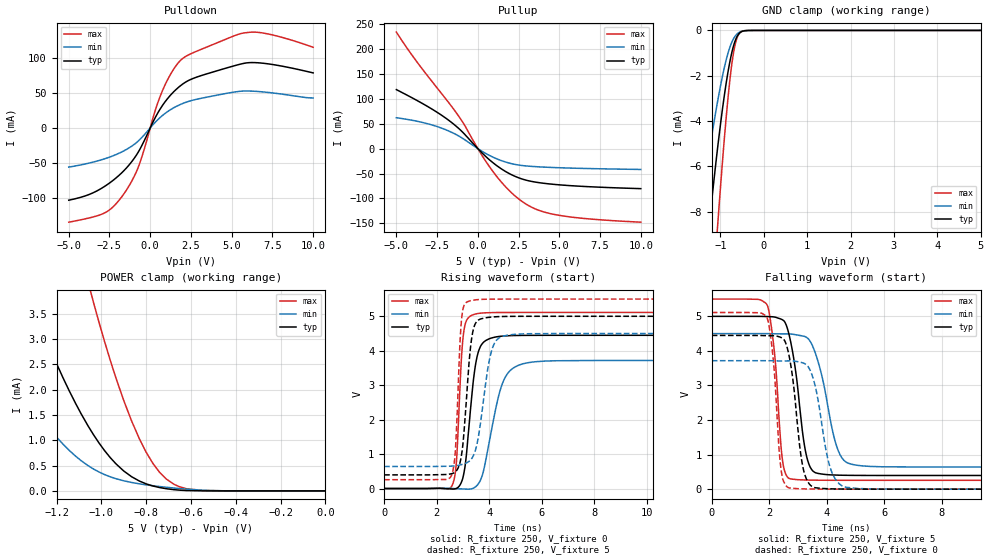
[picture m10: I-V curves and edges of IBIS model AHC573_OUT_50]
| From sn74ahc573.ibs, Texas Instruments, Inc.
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[Model]   AHC573_OUT_50
Model_type  3-state
Enable   Active-Low
Vref =   0.0
Rref =   1000
Cref =   50p
Vmeas =   2.5
| variable   typ   min   max
C_comp   2.10pF   1.84pF   2.26pF
| C_pullup   3.24pF   1.95pF   4.10pF
| C_pulldown   2.37pF   1.77pF   2.97pF
| C_tri-state   2.10pF   1.84pF   2.26pF
[Temperature Range]   40   100   -40
| Ambient temperature   25   85   -40
[Voltage range]   5   4.5   5.5
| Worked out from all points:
|   slope of the pulldown table from 0 to 0.75 V, typ, clamps not added: 23.5 ohm
|   slope of the pullup table from 0 to 0.75 V, typ, clamps not added: 32 ohm
|   GND clamp passes 1 mA (typ) near -0.74 V on its own axis
|   POWER clamp passes 1 mA (typ) near -1.02 V on its own axis
|   rising waveform, R_fixture 250, V_fixture 0: 20-80 % time 352ps typ, 620ps min, 198ps max; typ from 0 V to 4.45 V
|   falling waveform, R_fixture 250, V_fixture 5: 20-80 % time 427ps typ, 600ps min, 291ps max; typ from 5 V to 0.396 V
|   rising waveform, R_fixture 250, V_fixture 5: 20-80 % time 283ps typ, 440ps min, 176ps max; typ from 0.396 V to 5 V
|   falling waveform, R_fixture 250, V_fixture 0: 20-80 % time 363ps typ, 477ps min, 257ps max; typ from 4.45 V to 0 V
[GND Clamp]
| AHC573_OUT_50
|   Voltage   I(typ)   I(min)   I(max)
-5V       -113.4mA   -74.55mA   -144mA
-1.5V     -13.43mA   -8.541mA   -21.28mA
-1.27V    -8.795mA   -5.502mA   -14.35mA
-1.245V   -8.325mA   -5.193mA   -13.62mA
-1.07V    -5.258mA   -3.179mA   -8.755mA
-1.05V    -4.935mA   -2.968mA   -8.227mA
-875mV    -2.416mA   -1.357mA   -3.998mA
-765mV    -1.214mA   -649.6uA   -1.901mA
-665mV    -483.2uA   -264uA     -658.5uA
-615mV    -261.2uA   -152.9uA   -319.9uA
-545mV    -91.09uA   -61.69uA   -92.75uA
5V        41.61nA    4.678uA    381.8nA
[POWER Clamp]
| AHC573_OUT_50
|   Voltage   I(typ)   I(min)   I(max)
-5V       96.37mA    61.09mA    155.9mA
-1.595V   7.508mA    3.875mA    16.25mA
-1.32V    3.818mA    1.757mA    9.35mA
-1.2V     2.518mA    1.064mA    6.763mA
-1.06V    1.29mA     502uA      4.143mA
-1.035V   1.111mA    433.1uA    3.726mA
-935mV    536.6uA    242.1uA    2.235mA
-865mV    281uA      167.1uA    1.384mA
-800mV    139.6uA    120.4uA    765.1uA
-710mV    43.55uA    72.39uA    235.1uA
-545mV    1.289uA    12.21uA    8.438uA
-84.45fV  41.61nA    2.419nA    581.8nA
[Pulldown]
| AHC573_OUT_50
|   Voltage   I(typ)   I(min)   I(max)
-5V       -102.6mA   -55.6mA    -133.8mA
-2.78V    -82.71mA   -43.68mA   -120.5mA
-1.61V    -60.55mA   -32.45mA   -93.44mA
-700mV    -32.97mA   -17.85mA   -53.73mA
310mV     14.74mA    8.08mA     24.97mA
805mV     33.71mA    18.69mA    55.77mA
1.445V    51.45mA    28.67mA    83.68mA
2.05V     63.23mA    35.24mA    99.64mA
5.195V    88.52mA    51.1mA     131.2mA
6.16V     92.81mA    52.32mA    135.9mA
7.59V     89.77mA    49.49mA    131.6mA
10V       78.15mA    42.57mA    114.5mA
[Pullup]
| AHC573_OUT_50
|   Voltage   I(typ)   I(min)   I(max)
-5V       118.3mA    61.85mA    233.6mA
-3.725V   96.33mA    54.83mA    173.3mA
-1.74V    55.61mA    34.63mA    90.14mA
-930mV    32.84mA    20.44mA    53.02mA
125mV     -4.276mA   -2.671mA   -6.772mA
890mV     -27.29mA   -16.57mA   -44.24mA
1.705V    -45.94mA   -26.95mA   -76.63mA
2.52V     -58.72mA   -33.01mA   -101.2mA
3.53V     -67.14mA   -36.14mA   -121mA
4.76V     -71.97mA   -38.08mA   -132.4mA
6.765V    -76.29mA   -39.95mA   -140.8mA
10V       -80.28mA   -41.8mA    -147.5mA
[Ramp]
| AHC573_OUT_50
| variable   typ   min   max
dV/dt_r   2.68/3.60E-10   2.24/6.25E-10   3.07/2.02E-10
dV/dt_f   2.76/4.31E-10   2.32/6.04E-10   3.15/2.91E-10
R_load = 250
[Rising Waveform]
| AHC573_OUT_50
R_fixture =   250
C_fixture =   0
L_fixture =   0
V_fixture =   0
V_fixture_min = 0
V_fixture_max = 0
|   Time   V(typ)   V(min)   V(max)
0s        811.7pV    1.306nV    499pV
2.575ns   -14.16mV   1.506mV    72.69mV
2.75ns    3.938mV    -4.718mV   768.6mV
2.93ns    167.2mV    -9.851mV   3.639V
3.04ns    469.8mV    -13.69mV   4.607V
3.41ns    3.231V     16mV       5.051V
3.615ns   4.037V     171.4mV    5.086V
4.56ns    4.428V     3.158V     5.11V
5.725ns   4.447V     3.679V     5.112V
50ns      4.448V     3.717V     5.112V
[Falling Waveform]
| AHC573_OUT_50
R_fixture =   250
C_fixture =   0
L_fixture =   0
V_fixture =   5
V_fixture_min = 4.5
V_fixture_max = 5.5
|   Time   V(typ)   V(min)   V(max)
0s        5V         4.5V       5.5V
1.935ns   4.994V     4.499V     5.315V
2.185ns   4.98V      4.496V     3.932V
2.465ns   4.898V     4.492V     817.7mV
2.795ns   4.061V     4.485V     288.9mV
3.205ns   1.38V      4.424V     266.4mV
3.43ns    631.9mV    4.27V      262.1mV
4.41ns    405.4mV    1.099V     256.8mV
5.215ns   397.7mV    675.4mV    256.2mV
50ns      395.9mV    639.5mV    256.1mV
[Rising Waveform]
| AHC573_OUT_50
R_fixture =   250
C_fixture =   0
L_fixture =   0
V_fixture =   5
V_fixture_min = 4.5
V_fixture_max = 5.5
|   Time   V(typ)   V(min)   V(max)
0s        395.9mV    639.5mV    256.1mV
2.55ns    427.5mV    649.9mV    362.2mV
2.705ns   480.7mV    659.9mV    1.052V
2.885ns   747.2mV    683.9mV    4.224V
2.965ns   1.08V      699.3mV    5.044V
3.265ns   3.942V     811.4mV    5.448V
3.445ns   4.745V     1.043V     5.475V
4.11ns    4.979V     4.053V     5.498V
4.9ns     4.998V     4.471V     5.5V
50ns      5V         4.5V       5.5V
[Falling Waveform]
| AHC573_OUT_50
R_fixture =   250
C_fixture =   0
L_fixture =   0
V_fixture =   0
V_fixture_min = 0
V_fixture_max = 0
|   Time   V(typ)   V(min)   V(max)
0s        4.448V     3.717V     5.112V
1.92ns    4.441V     3.717V     4.966V
2.145ns   4.44V      3.714V     3.716V
2.41ns    4.389V     3.709V     585.9mV
2.71ns    3.781V     3.712V     32.25mV
3.19ns    571.2mV    3.647V     8.502mV
3.725ns   30.61mV    2.457V     2.673mV
4.21ns    8.435mV    430.9mV    1.019mV
5.06ns    1.522mV    21.89mV    204.3uV
50ns      1.364nV    4.471nV    592.4pV
